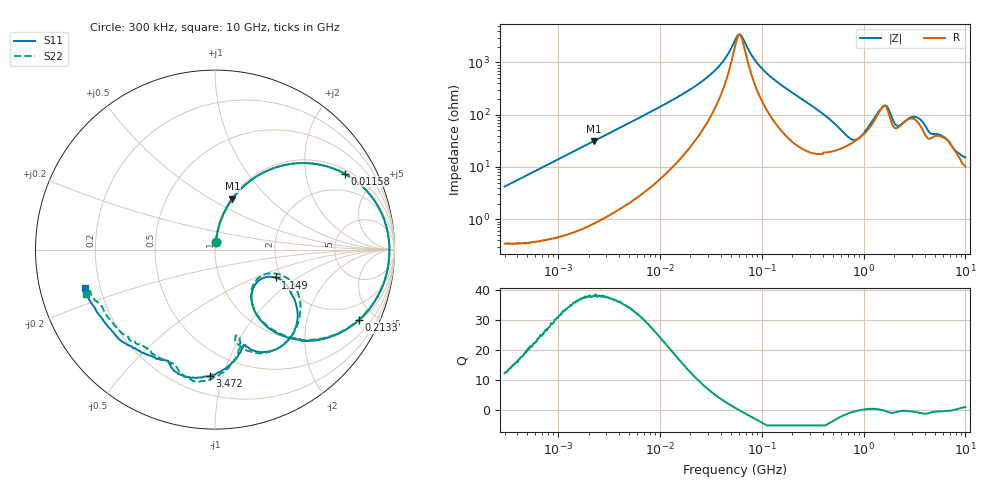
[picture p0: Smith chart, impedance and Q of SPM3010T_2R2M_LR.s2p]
! S-Parameter Data Generated by TDK Corporation
! Copyright(C) 2019 TDK Corporation.
! All Rights Reserved.
! TDK P/N: SPM3010T-2R2M-LR (Inductor)
! Property: L=2.2uH at 100kHz
! Size(LxWxT): 3.2x3x1mm
! Model Type: s2p (Touchstone File Format Version 1.0)
! Frequency: DC=Yes Start=0.3MHz Stop=10000MHz 802points Log-sweep
! Model Generated on Sep. 23, 2019
! Port Assignments:
!  1 ---@@@--- 2
! Applicable Conditions:
!  Temperature = 25 degC
!  DC Bias Current = 0 A
!  Small Signal Operation
! Terms and conditions regarding TDK Simulation Models
! (1)This simulation model is being provided solely for informational purposes. Please refer to the specifications of the products in terms of detailed characteristics of such products.
! (2)In no event shall TDK Corporation of any of its subsidiaries be liable for any loss or damage arising, directly or indirectly,
!  From any information contained in this simulation model, including, but not limited to loss or damages arising from any inaccuracies, omissions or errors in connection with such information.
! (3)Any and all copyrights on this simulation model are owned by TDK Corporation.
!  Duplication or redistribution of this simulation model without prior written permission from TDK Corporation is prohibited.
! (4)This simulation model is subject to any modification or change without any prior notice.
! (5)Neither TDK Corporation nor any of its subsidiaries shall make any warranty, express or implied,
!  Including but not limited to the correctness, implied warranties of merchantability and fitness for a particular purpose with respect to this simulation models.
! (6)The use of this simulation model shall be deemed to have consented to the terms and conditions hereof.
# Hz S MA R 50
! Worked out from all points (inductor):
!   801 points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, 300 kHz to 10 GHz, reference 50 ohm
!   read as one part in series: L = 2.23 uH near 318.3 kHz
!   highest Q = 38 at 2.276 MHz (marker M1), where L = 2.21 uH
!   self-resonance near 60.68 MHz
!   S11 on the Smith chart (normalised r, x): 300 kHz: 1.01, +0.09; 11.58 MHz: 1.17, +3.31; 213.3 MHz: 1.05, -4.08; 1.149 GHz: 1.86, -0.67; 3.472 GHz: 0.32, -0.90; 10 GHz: 0.14, -0.14
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300000  0.04294 83.0  0.9957 -2.4  0.9956 -2.3  0.04284 83.3
1713600  0.2306 75.1  0.9668 -13.3  0.9669 -13.3  0.2305 75.1
2275813  0.2991 71.1  0.9462 -17.4  0.9465 -17.4  0.2991 71.1
9671944  0.7902 35.3  0.5818 -52.4  0.5821 -52.3  0.7901 35.3
1.158341e7  0.8375 30.3  0.5093 -57.0  0.5097 -57.0  0.8374 30.3
3.206042e7  0.9618 8.3  0.1589 -72.4  0.159 -72.4  0.9617 8.3
5.477226e7  0.9717 0.1  0.0366 -40.2  0.03662 -40.2  0.9716 0.1
6.312136e7  0.9715 -2.0  0.02983 15.9  0.02983 15.9  0.9713 -1.9
1.050124e8  0.9612 -10.1  0.1361 67.3  0.1362 67.2  0.961 -9.9
2.133243e8  0.8936 -26.0  0.361 57.8  0.3611 57.8  0.8927 -25.8
3.126428e8  0.7956 -38.2  0.5169 45.0  0.5171 45.0  0.7939 -38.0
4.627802e8  0.6173 -51.5  0.6652 26.7  0.6654 26.7  0.6141 -51.1
6.738867e8  0.397 -56.9  0.7444 5.1  0.7446 5.1  0.3913 -56.6
8.987251e8  0.2967 -40.6  0.7196 -12.9  0.7199 -12.9  0.2868 -40.0
1.149233e9  0.3715 -24.7  0.6142 -28.8  0.6144 -28.8  0.3563 -21.9
1.481453e9  0.5406 -33.6  0.4076 -33.1  0.4078 -33.1  0.5801 -34.9
1.767019e9  0.6527 -54.1  0.393 -12.7  0.3931 -12.8  0.6485 -60.3
1.990462e9  0.6067 -68.6  0.5098 -16.5  0.5097 -16.6  0.5634 -74.8
2.355454e9  0.556 -73.2  0.5043 -32.6  0.5045 -32.7  0.4979 -74.9
3.472057e9  0.7037 -92.5  0.3871 -34.5  0.3875 -34.5  0.7068 -89.5
6.899057e9  0.7118 -130.7  0.3997 -66.0  0.3997 -66.0  0.6794 -128.8
1e10  0.7542 -163.5  0.337 -96.3  0.3375 -96.5  0.7594 -161.0
